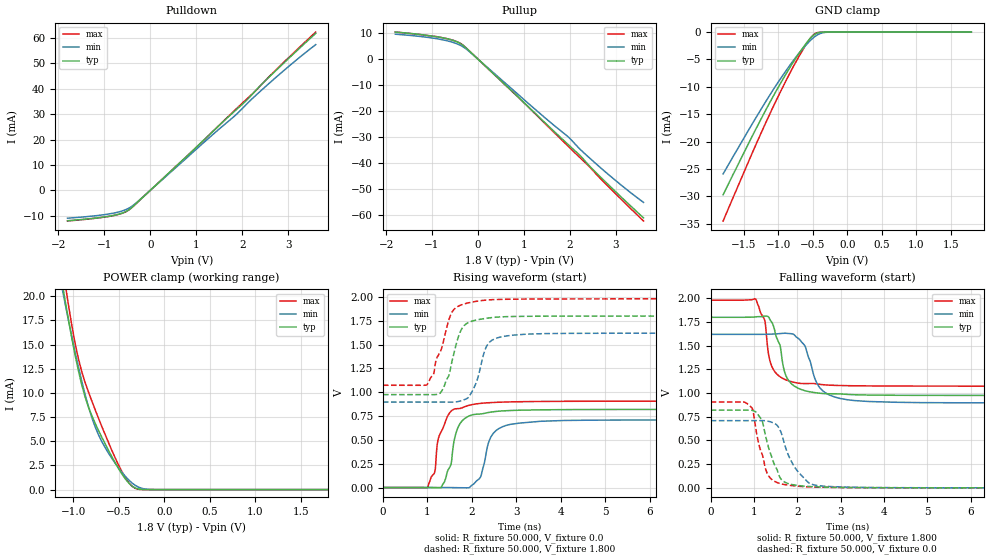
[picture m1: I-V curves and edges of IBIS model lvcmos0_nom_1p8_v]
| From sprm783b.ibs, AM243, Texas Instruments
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|   nom_1p8_v
[Model]   lvcmos0_nom_1p8_v
Model_type I/O
Polarity   Non-Inverting
Enable   Active-High
Vinl = 0
Vinh = 0.8
Vmeas = 0.9
Vref = 1.8
Cref = 2pF
Rref = 100000
|   typ   min   max
C_comp   5.313pF   5.138pF   5.385pF
[Voltage Range]   1.8   1.62   1.98
[Temperature Range]   27   150   -40
[Pullup Reference]   1.8   1.62   1.98
[Pulldown Reference]   0   0   0
[Power Clamp Reference]   1.8   1.62   1.98
[GND Clamp Reference]   0   0   0
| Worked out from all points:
|   slope of the pulldown table from 0 to 0.27 V, typ, clamps not added: 59.3 ohm
|   slope of the pullup table from 0 to 0.27 V, typ, clamps not added: 60 ohm
|   GND clamp passes 1 mA (typ) near -0.52 V on its own axis
|   POWER clamp passes 1 mA (typ) near -0.42 V on its own axis
|   rising waveform, R_fixture 50.000, V_fixture 0.0: 20-80 % time 268ps typ, 262ps min, 259ps max; typ from 0 V to 0.82 V
|   rising waveform, R_fixture 50.000, V_fixture 1.800: 20-80 % time 301ps typ, 282ps min, 348ps max; typ from 0.975 V to 1.8 V
|   falling waveform, R_fixture 50.000, V_fixture 1.800: 20-80 % time 298ps typ, 353ps min, 223ps max; typ from 1.8 V to 0.975 V
|   falling waveform, R_fixture 50.000, V_fixture 0.0: 20-80 % time 335ps typ, 434ps min, 272ps max; typ from 0.82 V to 0 V
[Pulldown]
|Voltage   I(typ)   I(min)   I(max)
-1.8V     -11.92mA   -10.93mA   -12.03mA
-1.194V   -10.89mA   -9.969mA   -10.95mA
-808mV    -9.857mA   -8.96mA    -9.935mA
-588mV    -8.778mA   -7.939mA   -8.877mA
-422mV    -7.06mA    -6.521mA   -7.099mA
-257mV    -4.345mA   -4.14mA    -4.333mA
955mV     16.15mA    15.41mA    16.09mA
1.837V    31.15mA    29.26mA    31.44mA
2.057V    34.72mA    33.17mA    35.2mA
2.278V    38.94mA    37.03mA    38.86mA
2.718V    46.83mA    44.15mA    47.05mA
3.6V      61.7mA     57.28mA    62.23mA
[Pullup]
|Voltage   I(typ)   I(min)   I(max)
-1.8V     10.47mA    9.652mA    10.48mA
-1.194V   9.383mA    8.634mA    9.35mA
-753mV    8.204mA    7.418mA    8.202mA
-478mV    6.836mA    6.068mA    6.907mA
-312mV    5.131mA    4.611mA    5.211mA
900mV     -15.03mA   -14.03mA   -15.13mA
1.947V    -32.72mA   -29.76mA   -33.34mA
2.222V    -37.22mA   -34.8mA    -38.07mA
2.443V    -41.56mA   -38.39mA   -41.85mA
2.718V    -46.41mA   -42.7mA    -47.08mA
3.214V    -54.86mA   -50mA      -55.8mA
3.6V      -61.24mA   -55.26mA   -62.44mA
[GND_clamp]
|Voltage   I(typ)   I(min)   I(max)
-1.8V     -29.72mA   -25.92mA   -34.52mA
-1.318V   -17.54mA   -15.51mA   -20.38mA
-1.132V   -13.09mA   -11.7mA    -15.22mA
-984mV    -9.729mA   -8.822mA   -11.3mA
-798mV    -5.797mA   -5.489mA   -6.696mA
-612mV    -2.352mA   -2.576mA   -2.564mA
-538mV    -1.179mA   -1.584mA   -1.166mA
-464mV    -369.8uA   -774.2uA   -275.4uA
-353mV    -16.01uA   -131.2uA   -4.376uA
-241mV    -388.4nA   -11.03uA   -119.1nA
1.8V      0A         0A         0A
[POWER_clamp]
|Voltage   I(typ)   I(min)   I(max)
-1.8V     63.47mA    56.87mA    71.37mA
-1.132V   21.93mA    21.28mA    24mA
-1.095V   19.86mA    19.49mA    21.65mA
-1.058V   17.85mA    17.74mA    19.39mA
-984mV    14.09mA    14.38mA    15.31mA
-909mV    10.91mA    11.3mA     12.26mA
-761mV    6.888mA    6.523mA    8.298mA
-649mV    4.716mA    4.333mA    5.678mA
-464mV    1.593mA    1.774mA    1.827mA
-315mV    150.2uA    416.6uA    111.8uA
-130mV    308.5nA    7.699uA    149nA
1.8V      0A         0A         0A
[Ramp]
| variable   typ   min   max
dV/dt_r   0.492/0.267n   0.426/0.263n   0.544/0.259n
dV/dt_f   0.495/0.298n   0.434/0.353n   0.544/0.223n
R_load = 50.000
[Rising Waveform]
R_fixture= 50.000
V_fixture= 0.0
|time   V(typ)   V(min)   V(max)
0s        815nV      17.91uV    1.383uV
1.005ns   106uV      16.08uV    1.636mV
1.171ns   -1.124mV   24.24uV    170.7mV
1.309ns   855.6uV    18.1uV     584.8mV
1.696ns   637.9mV    -1.709mV   828.1mV
2ns       761.7mV    24.35mV    869.8mV
2.195ns   772.2mV    109.5mV    883.1mV
2.427ns   791.7mV    530mV      891.3mV
2.86ns    808.2mV    662.3mV    898.7mV
10ns      819.8mV    709.6mV    906.4mV
[Rising Waveform]
R_fixture= 50.000
V_fixture= 1.800
V_fixture_min= 1.620
V_fixture_max= 1.980
|time   V(typ)   V(min)   V(max)
0s        975.3mV    896.8mV    1.073V
991ps     975.3mV    896.8mV    1.078V
1.283ns   988.9mV    896.7mV    1.417V
1.482ns   1.174V     896.7mV    1.757V
1.56ns    1.337V     896.7mV    1.845V
1.769ns   1.662V     911.5mV    1.918V
2.001ns   1.746V     1.003V     1.946V
2.328ns   1.776V     1.479V     1.968V
2.694ns   1.792V     1.584V     1.975V
10ns      1.8V       1.62V      1.98V
[Falling Waveform]
R_fixture= 50.000
V_fixture= 1.800
V_fixture_min= 1.620
V_fixture_max= 1.980
|time   V(typ)   V(min)   V(max)
0s        1.8V       1.62V      1.98V
1.041ns   1.804V     1.62V      1.99V
1.253ns   1.814V     1.621V     1.756V
1.331ns   1.805V     1.622V     1.421V
1.599ns   1.505V     1.628V     1.173V
1.738ns   1.182V     1.631V     1.139V
1.975ns   1.062V     1.592V     1.108V
2.483ns   1V         1.079V     1.095V
2.981ns   991.9mV    943.9mV    1.08V
10ns      975.3mV    896.8mV    1.073V
[Falling Waveform]
R_fixture= 50.000
V_fixture= 0.0
V_fixture_min= 0.0
V_fixture_max= 0.0
|time   V(typ)   V(min)   V(max)
0s        819.8mV    709.6mV    906.4mV
837ps     819.8mV    709.6mV    890.7mV
968ps     815.9mV    709.6mV    827.7mV
1.051ns   796.4mV    709.6mV    599.9mV
1.185ns   709.5mV    709.7mV    356.3mV
1.313ns   465.1mV    704.2mV    145.5mV
1.662ns   74.28mV    530.1mV    38.6mV
1.961ns   28.16mV    202.4mV    19.29mV
2.459ns   10.02mV    25.31mV    7.547mV
10ns      42.39uV    105uV      26.07uV
